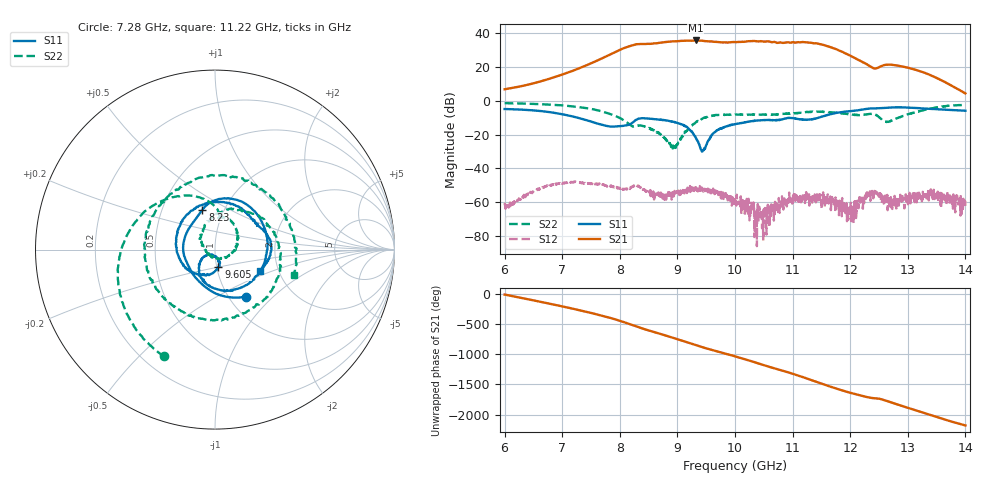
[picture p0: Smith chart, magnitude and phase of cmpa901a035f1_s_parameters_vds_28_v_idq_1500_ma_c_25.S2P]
!Keysight Technologies,E5071C,MY46110325,B.14.03
!Date: Wed Mar 10 10:58:39 2021
!Data & Calibration Information:
!Freq	S11:SOLT2(ON)	S21:SOLT2(ON)	S12:SOLT2(ON)	S22:SOLT2(ON)
!PortZ  Port1:50+j0  Port2:50+j0
!Above PortZ is port z conversion or system Z0 setting when saving the data.
!When reading, reference impedance value at option line is always used.
# Hz S dB R 50
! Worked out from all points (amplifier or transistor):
!   1601 points, 6 GHz to 14 GHz, reference 50 ohm
!   highest |S21| = 35.8 dB at 9.32 GHz (marker M1)
!   |S21| within 3 dB of that: 8.207 GHz to 11.57 GHz (3.359 GHz wide, 34 % of centre)
!   unconditionally stable (mu >= 1): start of sweep to end of sweep
!   at 7.33 GHz: K = 7.49, MAG = 22.5 dB, |S12| = -48.6 dB
!   at 10 GHz: K = 6.42, MAG = 35.8 dB, |S12| = -58.8 dB
!   at 14 GHz: K = 120.43, MAG = 9.5 dB, |S12| = -62.1 dB
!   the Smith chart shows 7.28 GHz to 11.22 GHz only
!   S11 on the Smith chart (normalised r, x): 7.28 GHz: 1.20, -0.70; 8.23 GHz: 0.79, +0.37; 9.605 GHz: 1.02, -0.20; 11.22 GHz: 1.60, -0.42
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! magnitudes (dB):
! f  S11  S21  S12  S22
! 6 GHz  -4.8  6.9  -61.5  -1.3
! 6.695 GHz  -6.3  12.3  -50.8  -2.0
! 7.28 GHz  -10.1  19.1  -48.1  -3.6
! 7.335 GHz  -10.6  19.9  -48.6  -3.9
! 7.845 GHz  -15.2  27.8  -50.6  -7.9
! 8.23 GHz  -12.6  33.1  -50.7  -15.1
! 8.67 GHz  -11.0  34.4  -54.2  -19.1
! 8.94 GHz  -12.5  35.3  -57.6  -27.2
! 9.32 GHz  -21.9  35.8  -52.5  -12.7
! 9.445 GHz  -29.5  35.6  -53.4  -10.2
! 9.605 GHz  -19.9  35.3  -52.7  -8.7
! 10 GHz  -13.9  34.9  -58.8  -8.1
! 10.51 GHz  -11.4  35.2  -68.6  -8.1
! 10.85 GHz  -10.7  34.4  -58.8  -7.7
! 11.22 GHz  -11.1  34.8  -55.8  -6.7
! 11.34 GHz  -10.9  34.4  -57.1  -6.4
! 11.62 GHz  -8.3  32.3  -57.1  -6.5
! 11.98 GHz  -6.1  27.1  -64.8  -7.9
! 12.4 GHz  -4.4  19.4  -55.0  -7.8
! 12.67 GHz  -4.0  21.5  -57.8  -12.4
! 13.38 GHz  -4.7  15.5  -56.1  -4.7
! 14 GHz  -5.8  4.5  -62.1  -2.4
